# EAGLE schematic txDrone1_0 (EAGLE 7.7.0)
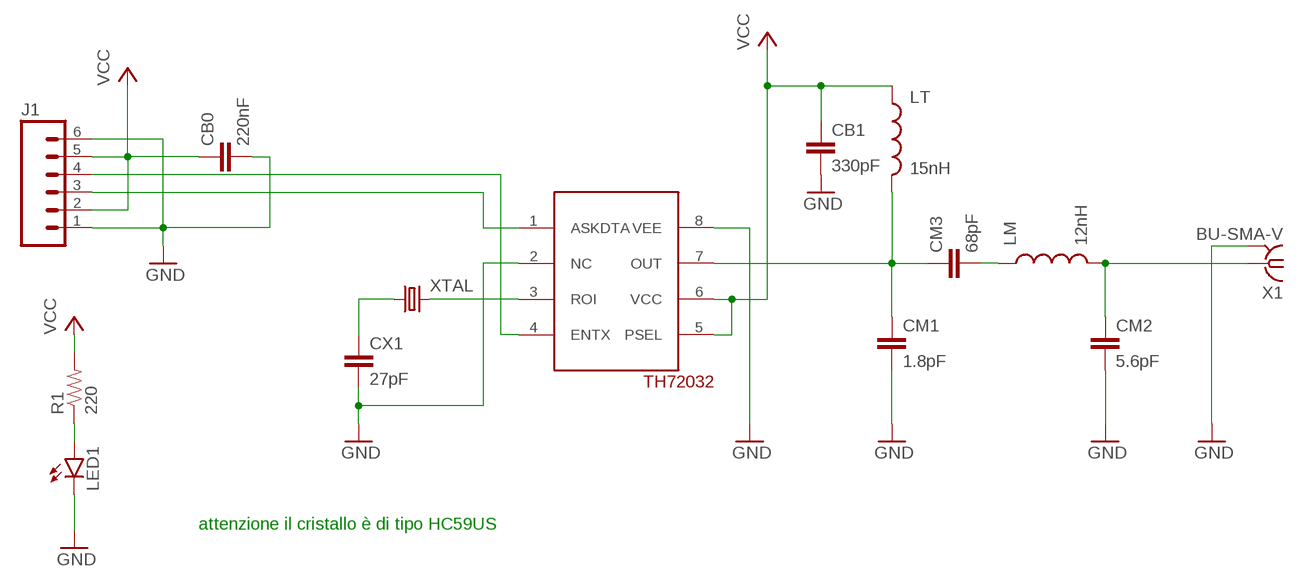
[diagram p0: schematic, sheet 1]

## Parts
CB0  220nF  2.2UF-25V-+80/-20(0805)  [0805-CAP]
CB1  330pF  2.2UF-25V-+80/-20(0805)  [0805-CAP]
CM1  1.8pF  2.2UF-25V-+80/-20(0805)  [0805-CAP]
CM2  5.6pF  2.2UF-25V-+80/-20(0805)  [0805-CAP]
CM3  68pF  2.2UF-25V-+80/-20(0805)  [0805-CAP]
CX1  27pF  2.2UF-25V-+80/-20(0805)  [0805-CAP]
J1  M063.5MM-6  [SCREWTERMINAL-3.5MM-6@1]
LED1  LED1206  [LED-1206]
LM  12nH  INDUCTOR0805  [0805]
LT  15nH  INDUCTOR0805  [0805]
R1  220  RESISTOR0805-RES  [0805]
U$1  TH72032NORMAL  [SO08]
X1  BU-SMA-V  [BU-SMA-V]
XTAL  CRYSTALHC49UV  [HC49U-V]

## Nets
GND: CB0.2 CB1.2 CM1.2 CM2.2 CX1.2 J1.1 J1.6 LED1.C U$1.2(NC) U$1.8(VEE) X1.2 X1.3 X1.4 X1.5
N$1: CM1.1 CM3.1 LT.2 U$1.7(OUT)
N$2: CM3.2 LM.1
N$3: CM2.1 LM.2 X1.1
N$4: U$1.3(ROI) XTAL.2
N$5: CX1.1 XTAL.1
N$6: J1.3 U$1.1(ASKDTA)
N$7: J1.4 U$1.4(ENTX)
N$8: LED1.A R1.1
VCC: CB0.1 CB1.1 J1.2 J1.5 LT.1 R1.2 U$1.5(PSEL) U$1.6(VCC)

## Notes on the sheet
- attenzione il cristallo è di tipo HC59US

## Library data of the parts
CB0 CB1 CM1-CM3 CX1 = SparkFun-Capacitors:2.2UF-25V-+80/-20(0805): CAP-11624; PROD_ID: CAP-11624; VALUE: 2.2uF
J1 = SparkFun-Connectors:M06: Header 6 Standard 6-pin 0.1" header. Use with straight break away headers (SKU : PRT-00116), right angle break away headers (PRT-00553), swiss pins (PRT-00743), machine pins (PRT-00117), and female headers (PRT-00115). Molex polarized connector foot print use with SKU : PRT-08094 with associated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
LED1 = SparkFun-LED:LED: LEDs
LM LT = SparkFun-Passives:INDUCTOR: Inductors
R1 = SparkFun-Resistors:RESISTOR: Resistor
U$1 = th72032:TH72032
X1 = con-coax:BU-SMA-V: FEMALE SMA CONNECTOR; OC_FARNELL: unknown; OC_NEWARK: unknown
XTAL = SparkFun-FreqCtrl:CRYSTAL: Various standard crystals. Proven footprints.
